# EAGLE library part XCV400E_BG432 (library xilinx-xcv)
xcv400e_bg432 edit this description Auto generated by make-symbol-device-package-bsdl.ulp Rev. 26 Source: xcv400e_bg432.bsd
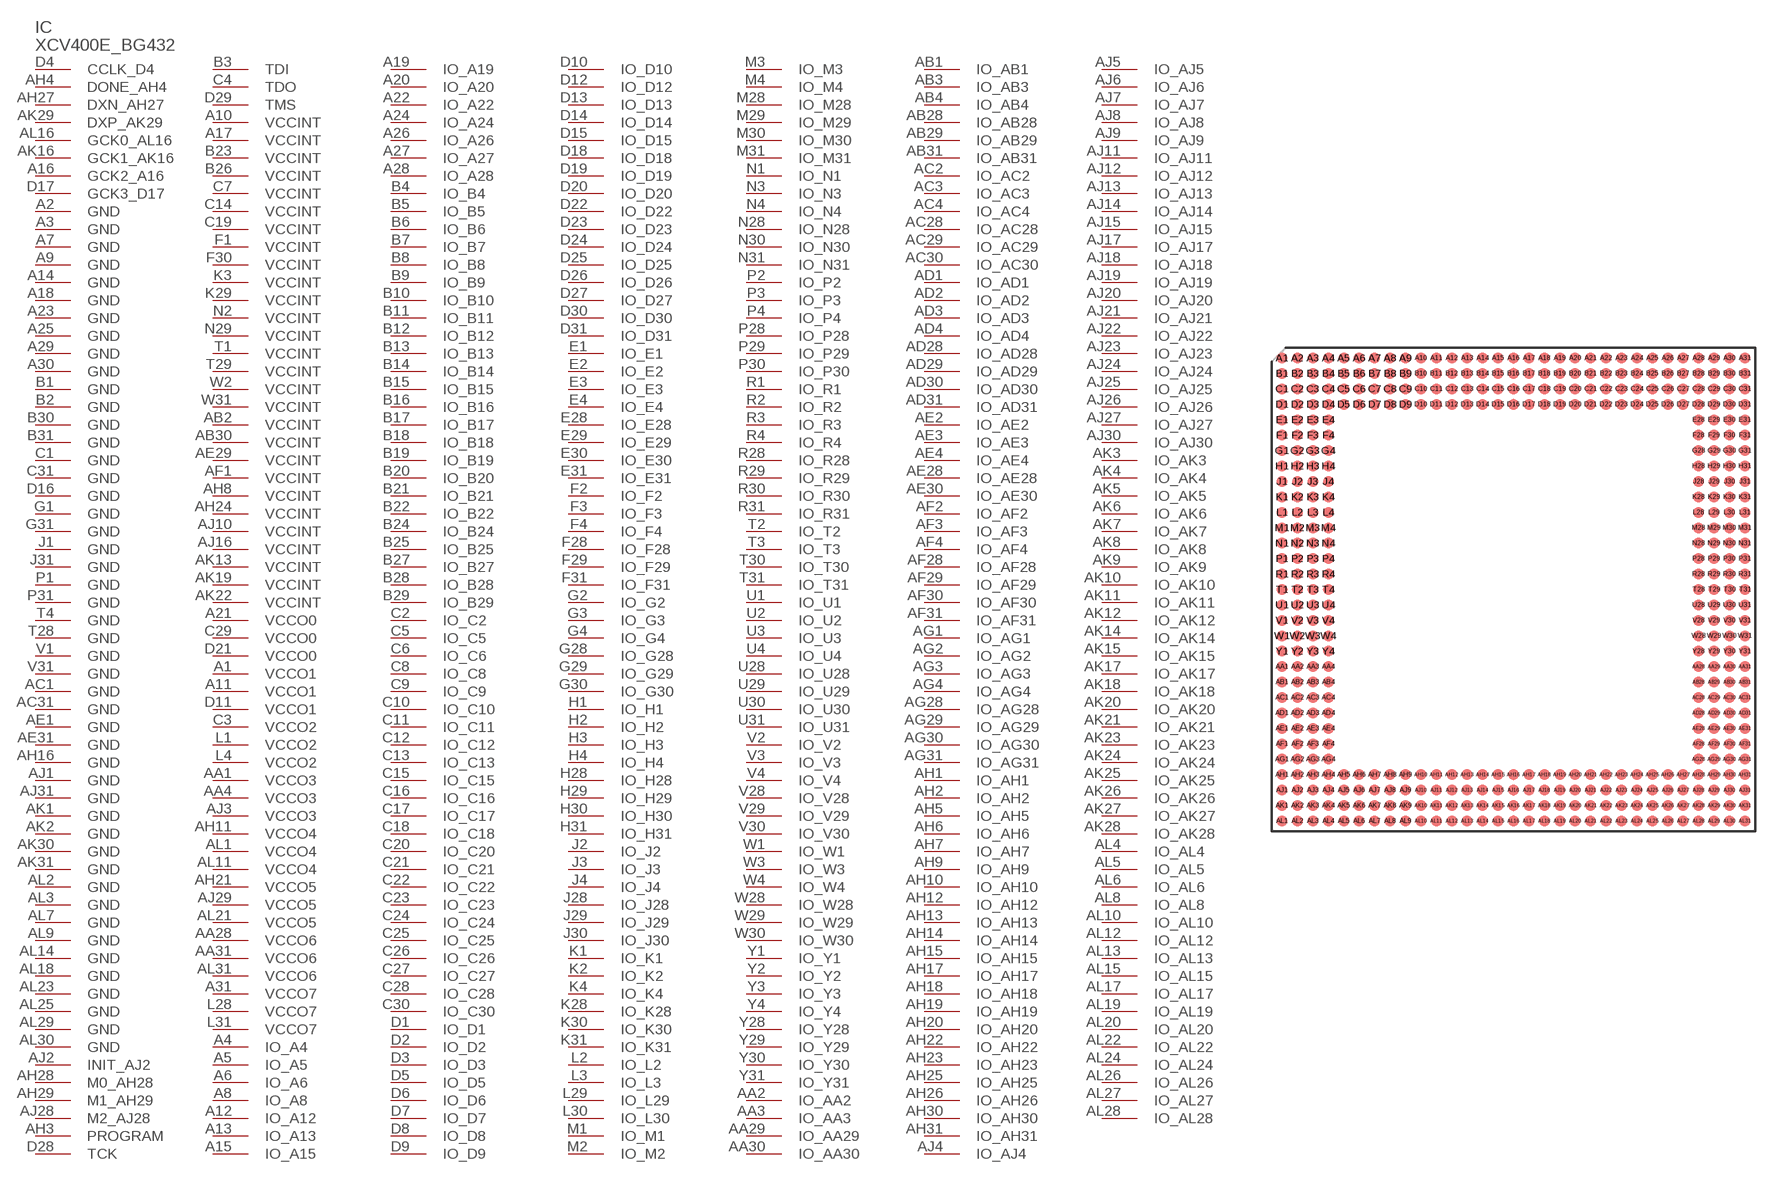
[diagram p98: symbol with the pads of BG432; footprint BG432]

Designator prefix IC

## XCV400E_BG432 (OC_FARNELL: unknown; OC_NEWARK: unknown)  [BG432]
A1  VCCO1  pwr
A2  GND  pwr
A3  GND  pwr
A4  IO_A4
A5  IO_A5
A6  IO_A6
A7  GND  pwr
A8  IO_A8
A9  GND  pwr
A10  VCCINT  pwr
A11  VCCO1  pwr
A12  IO_A12
A13  IO_A13
A14  GND  pwr
A15  IO_A15
A16  GCK2_A16  in
A17  VCCINT  pwr
A18  GND  pwr
A19  IO_A19
A20  IO_A20
A21  VCCO0  pwr
A22  IO_A22
A23  GND  pwr
A24  IO_A24
A25  GND  pwr
A26  IO_A26
A27  IO_A27
A28  IO_A28
A29  GND  pwr
A30  GND  pwr
A31  VCCO7  pwr
AA1  VCCO3  pwr
AA2  IO_AA2
AA3  IO_AA3
AA4  VCCO3  pwr
AA28  VCCO6  pwr
AA29  IO_AA29
AA30  IO_AA30
AA31  VCCO6  pwr
AB1  IO_AB1
AB2  VCCINT  pwr
AB3  IO_AB3
AB4  IO_AB4
AB28  IO_AB28
AB29  IO_AB29
AB30  VCCINT  pwr
AB31  IO_AB31
AC1  GND  pwr
AC2  IO_AC2
AC3  IO_AC3
AC4  IO_AC4
AC28  IO_AC28
AC29  IO_AC29
AC30  IO_AC30
AC31  GND  pwr
AD1  IO_AD1
AD2  IO_AD2
AD3  IO_AD3
AD4  IO_AD4
AD28  IO_AD28
AD29  IO_AD29
AD30  IO_AD30
AD31  IO_AD31
AE1  GND  pwr
AE2  IO_AE2
AE3  IO_AE3
AE4  IO_AE4
AE28  IO_AE28
AE29  VCCINT  pwr
AE30  IO_AE30
AE31  GND  pwr
AF1  VCCINT  pwr
AF2  IO_AF2
AF3  IO_AF3
AF4  IO_AF4
AF28  IO_AF28
AF29  IO_AF29
AF30  IO_AF30
AF31  IO_AF31
AG1  IO_AG1
AG2  IO_AG2
AG3  IO_AG3
AG4  IO_AG4
AG28  IO_AG28
AG29  IO_AG29
AG30  IO_AG30
AG31  IO_AG31
AH1  IO_AH1
AH2  IO_AH2
AH3  PROGRAM  in
AH4  DONE_AH4
AH5  IO_AH5
AH6  IO_AH6
AH7  IO_AH7
AH8  VCCINT  pwr
AH9  IO_AH9
AH10  IO_AH10
AH11  VCCO4  pwr
AH12  IO_AH12
AH13  IO_AH13
AH14  IO_AH14
AH15  IO_AH15
AH16  GND  pwr
AH17  IO_AH17
AH18  IO_AH18
AH19  IO_AH19
AH20  IO_AH20
AH21  VCCO5  pwr
AH22  IO_AH22
AH23  IO_AH23
AH24  VCCINT  pwr
AH25  IO_AH25
AH26  IO_AH26
AH27  DXN_AH27  pas
AH28  M0_AH28  in
AH29  M1_AH29  in
AH30  IO_AH30
AH31  IO_AH31
AJ1  GND  pwr
AJ2  INIT_AJ2
AJ3  VCCO3  pwr
AJ4  IO_AJ4
AJ5  IO_AJ5
AJ6  IO_AJ6
AJ7  IO_AJ7
AJ8  IO_AJ8
AJ9  IO_AJ9
AJ10  VCCINT  pwr
AJ11  IO_AJ11
AJ12  IO_AJ12
AJ13  IO_AJ13
AJ14  IO_AJ14
AJ15  IO_AJ15
AJ16  VCCINT  pwr
AJ17  IO_AJ17
AJ18  IO_AJ18
AJ19  IO_AJ19
AJ20  IO_AJ20
AJ21  IO_AJ21
AJ22  IO_AJ22
AJ23  IO_AJ23
AJ24  IO_AJ24
AJ25  IO_AJ25
AJ26  IO_AJ26
AJ27  IO_AJ27
AJ28  M2_AJ28  in
AJ29  VCCO5  pwr
AJ30  IO_AJ30
AJ31  GND  pwr
AK1  GND  pwr
AK2  GND  pwr
AK3  IO_AK3
AK4  IO_AK4
AK5  IO_AK5
AK6  IO_AK6
AK7  IO_AK7
AK8  IO_AK8
AK9  IO_AK9
AK10  IO_AK10
AK11  IO_AK11
AK12  IO_AK12
AK13  VCCINT  pwr
AK14  IO_AK14
AK15  IO_AK15
AK16  GCK1_AK16  in
AK17  IO_AK17
AK18  IO_AK18
AK19  VCCINT  pwr
AK20  IO_AK20
AK21  IO_AK21
AK22  VCCINT  pwr
AK23  IO_AK23
AK24  IO_AK24
AK25  IO_AK25
AK26  IO_AK26
AK27  IO_AK27
AK28  IO_AK28
AK29  DXP_AK29  pas
AK30  GND  pwr
AK31  GND  pwr
AL1  VCCO4  pwr
AL2  GND  pwr
AL3  GND  pwr
AL4  IO_AL4
AL5  IO_AL5
AL6  IO_AL6
AL7  GND  pwr
AL8  IO_AL8
AL9  GND  pwr
AL10  IO_AL10
AL11  VCCO4  pwr
AL12  IO_AL12
AL13  IO_AL13
AL14  GND  pwr
AL15  IO_AL15
AL16  GCK0_AL16  in
AL17  IO_AL17
AL18  GND  pwr
AL19  IO_AL19
AL20  IO_AL20
AL21  VCCO5  pwr
AL22  IO_AL22
AL23  GND  pwr
AL24  IO_AL24
AL25  GND  pwr
AL26  IO_AL26
AL27  IO_AL27
AL28  IO_AL28
AL29  GND  pwr
AL30  GND  pwr
AL31  VCCO6  pwr
B1  GND  pwr
B2  GND  pwr
B3  TDI  in
B4  IO_B4
B5  IO_B5
B6  IO_B6
B7  IO_B7
B8  IO_B8
B9  IO_B9
B10  IO_B10
B11  IO_B11
B12  IO_B12
B13  IO_B13
B14  IO_B14
B15  IO_B15
B16  IO_B16
B17  IO_B17
B18  IO_B18
B19  IO_B19
B20  IO_B20
B21  IO_B21
B22  IO_B22
B23  VCCINT  pwr
B24  IO_B24
B25  IO_B25
B26  VCCINT  pwr
B27  IO_B27
B28  IO_B28
B29  IO_B29
B30  GND  pwr
B31  GND  pwr
C1  GND  pwr
C2  IO_C2
C3  VCCO2  pwr
C4  TDO  out
C5  IO_C5
C6  IO_C6
C7  VCCINT  pwr
C8  IO_C8
C9  IO_C9
C10  IO_C10
C11  IO_C11
C12  IO_C12
C13  IO_C13
C14  VCCINT  pwr
C15  IO_C15
C16  IO_C16
C17  IO_C17
C18  IO_C18
C19  VCCINT  pwr
C20  IO_C20
C21  IO_C21
C22  IO_C22
C23  IO_C23
C24  IO_C24
C25  IO_C25
C26  IO_C26
C27  IO_C27
C28  IO_C28
C29  VCCO0  pwr
C30  IO_C30
C31  GND  pwr
D1  IO_D1
D2  IO_D2
D3  IO_D3
D4  CCLK_D4
D5  IO_D5
D6  IO_D6
D7  IO_D7
D8  IO_D8
D9  IO_D9
D10  IO_D10
D11  VCCO1  pwr
D12  IO_D12
D13  IO_D13
D14  IO_D14
D15  IO_D15
D16  GND  pwr
D17  GCK3_D17  in
D18  IO_D18
D19  IO_D19
D20  IO_D20
D21  VCCO0  pwr
D22  IO_D22
D23  IO_D23
D24  IO_D24
D25  IO_D25
D26  IO_D26
D27  IO_D27
D28  TCK  in
D29  TMS  in
D30  IO_D30
D31  IO_D31
E1  IO_E1
E2  IO_E2
E3  IO_E3
E4  IO_E4
E28  IO_E28
E29  IO_E29
E30  IO_E30
E31  IO_E31
F1  VCCINT  pwr
F2  IO_F2
F3  IO_F3
F4  IO_F4
F28  IO_F28
F29  IO_F29
F30  VCCINT  pwr
F31  IO_F31
G1  GND  pwr
G2  IO_G2
G3  IO_G3
G4  IO_G4
G28  IO_G28
G29  IO_G29
G30  IO_G30
G31  GND  pwr
H1  IO_H1
H2  IO_H2
H3  IO_H3
H4  IO_H4
H28  IO_H28
H29  IO_H29
H30  IO_H30
H31  IO_H31
J1  GND  pwr
J2  IO_J2
J3  IO_J3
J4  IO_J4
J28  IO_J28
J29  IO_J29
J30  IO_J30
J31  GND  pwr
K1  IO_K1
K2  IO_K2
K3  VCCINT  pwr
K4  IO_K4
K28  IO_K28
K29  VCCINT  pwr
K30  IO_K30
K31  IO_K31
L1  VCCO2  pwr
L2  IO_L2
L3  IO_L3
L4  VCCO2  pwr
L28  VCCO7  pwr
L29  IO_L29
L30  IO_L30
L31  VCCO7  pwr
M1  IO_M1
M2  IO_M2
M3  IO_M3
M4  IO_M4
M28  IO_M28
M29  IO_M29
M30  IO_M30
M31  IO_M31
N1  IO_N1
N2  VCCINT  pwr
N3  IO_N3
N4  IO_N4
N28  IO_N28
N29  VCCINT  pwr
N30  IO_N30
N31  IO_N31
P1  GND  pwr
P2  IO_P2
P3  IO_P3
P4  IO_P4
P28  IO_P28
P29  IO_P29
P30  IO_P30
P31  GND  pwr
R1  IO_R1
R2  IO_R2
R3  IO_R3
R4  IO_R4
R28  IO_R28
R29  IO_R29
R30  IO_R30
R31  IO_R31
T1  VCCINT  pwr
T2  IO_T2
T3  IO_T3
T4  GND  pwr
T28  GND  pwr
T29  VCCINT  pwr
T30  IO_T30
T31  IO_T31
U1  IO_U1
U2  IO_U2
U3  IO_U3
U4  IO_U4
U28  IO_U28
U29  IO_U29
U30  IO_U30
U31  IO_U31
V1  GND  pwr
V2  IO_V2
V3  IO_V3
V4  IO_V4
V28  IO_V28
V29  IO_V29
V30  IO_V30
V31  GND  pwr
W1  IO_W1
W2  VCCINT  pwr
W3  IO_W3
W4  IO_W4
W28  IO_W28
W29  IO_W29
W30  IO_W30
W31  VCCINT  pwr
Y1  IO_Y1
Y2  IO_Y2
Y3  IO_Y3
Y4  IO_Y4
Y28  IO_Y28
Y29  IO_Y29
Y30  IO_Y30
Y31  IO_Y31

## Footprint BG432 (pad centres in mm)
xcv300_bg432 edit this description Auto generated by make-symbol-device-package-bsdl.ulp Rev. 26 Source: xcv300_bg432.bsd
smd 0.9 x 0.9: A1 -19.05,19.05; A2 -17.78,19.05; A3 -16.51,19.05; A4 -15.24,19.05; A5 -13.97,19.05; A6 -12.7,19.05; A7 -11.43,19.05; A8 -10.16,19.05; A9 -8.89,19.05; A10 -7.62,19.05; A11 -6.35,19.05; A12 -5.08,19.05; A13 -3.81,19.05; A14 -2.54,19.05; A15 -1.27,19.05; A16 0,19.05; A17 1.27,19.05; A18 2.54,19.05; A19 3.81,19.05; A20 5.08,19.05; A21 6.35,19.05; A22 7.62,19.05; A23 8.89,19.05; A24 10.16,19.05; A25 11.43,19.05; A26 12.7,19.05; A27 13.97,19.05; A28 15.24,19.05; A29 16.51,19.05; A30 17.78,19.05; A31 19.05,19.05; AA1 -19.05,-6.35; AA2 -17.78,-6.35; AA3 -16.51,-6.35; AA4 -15.24,-6.35; AA28 15.24,-6.35; AA29 16.51,-6.35; AA30 17.78,-6.35; AA31 19.05,-6.35; AB1 -19.05,-7.62; AB2 -17.78,-7.62; AB3 -16.51,-7.62; AB4 -15.24,-7.62; AB28 15.24,-7.62; AB29 16.51,-7.62; AB30 17.78,-7.62; AB31 19.05,-7.62; AC1 -19.05,-8.89; AC2 -17.78,-8.89; AC3 -16.51,-8.89; AC4 -15.24,-8.89; AC28 15.24,-8.89; AC29 16.51,-8.89; AC30 17.78,-8.89; AC31 19.05,-8.89; AD1 -19.05,-10.16; AD2 -17.78,-10.16; AD3 -16.51,-10.16; AD4 -15.24,-10.16; AD28 15.24,-10.16; AD29 16.51,-10.16; AD30 17.78,-10.16; AD31 19.05,-10.16; AE1 -19.05,-11.43; AE2 -17.78,-11.43; AE3 -16.51,-11.43; AE4 -15.24,-11.43; AE28 15.24,-11.43; AE29 16.51,-11.43; AE30 17.78,-11.43; AE31 19.05,-11.43; AF1 -19.05,-12.7; AF2 -17.78,-12.7; AF3 -16.51,-12.7; AF4 -15.24,-12.7; AF28 15.24,-12.7; AF29 16.51,-12.7; AF30 17.78,-12.7; AF31 19.05,-12.7; AG1 -19.05,-13.97; AG2 -17.78,-13.97; AG3 -16.51,-13.97; AG4 -15.24,-13.97; AG28 15.24,-13.97; AG29 16.51,-13.97; AG30 17.78,-13.97; AG31 19.05,-13.97; AH1 -19.05,-15.24; AH2 -17.78,-15.24; AH3 -16.51,-15.24; AH4 -15.24,-15.24; AH5 -13.97,-15.24; AH6 -12.7,-15.24; AH7 -11.43,-15.24; AH8 -10.16,-15.24; AH9 -8.89,-15.24; AH10 -7.62,-15.24; AH11 -6.35,-15.24; AH12 -5.08,-15.24; AH13 -3.81,-15.24; AH14 -2.54,-15.24; AH15 -1.27,-15.24; AH16 0,-15.24; AH17 1.27,-15.24; AH18 2.54,-15.24; AH19 3.81,-15.24; AH20 5.08,-15.24; AH21 6.35,-15.24; AH22 7.62,-15.24; AH23 8.89,-15.24; AH24 10.16,-15.24; AH25 11.43,-15.24; AH26 12.7,-15.24; AH27 13.97,-15.24; AH28 15.24,-15.24; AH29 16.51,-15.24; AH30 17.78,-15.24; AH31 19.05,-15.24; AJ1 -19.05,-16.51; AJ2 -17.78,-16.51; AJ3 -16.51,-16.51; AJ4 -15.24,-16.51; AJ5 -13.97,-16.51; AJ6 -12.7,-16.51; AJ7 -11.43,-16.51; AJ8 -10.16,-16.51; AJ9 -8.89,-16.51; AJ10 -7.62,-16.51; AJ11 -6.35,-16.51; AJ12 -5.08,-16.51; AJ13 -3.81,-16.51; AJ14 -2.54,-16.51; AJ15 -1.27,-16.51; AJ16 0,-16.51; AJ17 1.27,-16.51; AJ18 2.54,-16.51; AJ19 3.81,-16.51; AJ20 5.08,-16.51; AJ21 6.35,-16.51; AJ22 7.62,-16.51; AJ23 8.89,-16.51; AJ24 10.16,-16.51; AJ25 11.43,-16.51; AJ26 12.7,-16.51; AJ27 13.97,-16.51; AJ28 15.24,-16.51; AJ29 16.51,-16.51; AJ30 17.78,-16.51; AJ31 19.05,-16.51; AK1 -19.05,-17.78; AK2 -17.78,-17.78; AK3 -16.51,-17.78; AK4 -15.24,-17.78; AK5 -13.97,-17.78; AK6 -12.7,-17.78; AK7 -11.43,-17.78; AK8 -10.16,-17.78; AK9 -8.89,-17.78; AK10 -7.62,-17.78; AK11 -6.35,-17.78; AK12 -5.08,-17.78; AK13 -3.81,-17.78; AK14 -2.54,-17.78; AK15 -1.27,-17.78; AK16 0,-17.78; AK17 1.27,-17.78; AK18 2.54,-17.78; AK19 3.81,-17.78; AK20 5.08,-17.78; AK21 6.35,-17.78; AK22 7.62,-17.78; AK23 8.89,-17.78; AK24 10.16,-17.78; AK25 11.43,-17.78; AK26 12.7,-17.78; AK27 13.97,-17.78; AK28 15.24,-17.78; AK29 16.51,-17.78; AK30 17.78,-17.78; AK31 19.05,-17.78; AL1 -19.05,-19.05; AL2 -17.78,-19.05; AL3 -16.51,-19.05; AL4 -15.24,-19.05; AL5 -13.97,-19.05; AL6 -12.7,-19.05; AL7 -11.43,-19.05; AL8 -10.16,-19.05; AL9 -8.89,-19.05; AL10 -7.62,-19.05; AL11 -6.35,-19.05; AL12 -5.08,-19.05; AL13 -3.81,-19.05; AL14 -2.54,-19.05; AL15 -1.27,-19.05; AL16 0,-19.05; AL17 1.27,-19.05; AL18 2.54,-19.05; AL19 3.81,-19.05; AL20 5.08,-19.05; AL21 6.35,-19.05; AL22 7.62,-19.05; AL23 8.89,-19.05; AL24 10.16,-19.05; AL25 11.43,-19.05; AL26 12.7,-19.05; AL27 13.97,-19.05; AL28 15.24,-19.05; AL29 16.51,-19.05; AL30 17.78,-19.05; AL31 19.05,-19.05; B1 -19.05,17.78; B2 -17.78,17.78; B3 -16.51,17.78; B4 -15.24,17.78; B5 -13.97,17.78; B6 -12.7,17.78; B7 -11.43,17.78; B8 -10.16,17.78; B9 -8.89,17.78; B10 -7.62,17.78; B11 -6.35,17.78; B12 -5.08,17.78; B13 -3.81,17.78; B14 -2.54,17.78; B15 -1.27,17.78; B16 0,17.78; B17 1.27,17.78; B18 2.54,17.78; B19 3.81,17.78; B20 5.08,17.78; B21 6.35,17.78; B22 7.62,17.78; B23 8.89,17.78; B24 10.16,17.78; B25 11.43,17.78; B26 12.7,17.78; B27 13.97,17.78; B28 15.24,17.78; B29 16.51,17.78; B30 17.78,17.78; B31 19.05,17.78; C1 -19.05,16.51; C2 -17.78,16.51; C3 -16.51,16.51; C4 -15.24,16.51; C5 -13.97,16.51; C6 -12.7,16.51; C7 -11.43,16.51; C8 -10.16,16.51; C9 -8.89,16.51; C10 -7.62,16.51; C11 -6.35,16.51; C12 -5.08,16.51; C13 -3.81,16.51; C14 -2.54,16.51; C15 -1.27,16.51; C16 0,16.51; C17 1.27,16.51; C18 2.54,16.51; C19 3.81,16.51; C20 5.08,16.51; C21 6.35,16.51; C22 7.62,16.51; C23 8.89,16.51; C24 10.16,16.51; C25 11.43,16.51; C26 12.7,16.51; C27 13.97,16.51; C28 15.24,16.51; C29 16.51,16.51; C30 17.78,16.51; C31 19.05,16.51; D1 -19.05,15.24; D2 -17.78,15.24; D3 -16.51,15.24; D4 -15.24,15.24; D5 -13.97,15.24; D6 -12.7,15.24; D7 -11.43,15.24; D8 -10.16,15.24; D9 -8.89,15.24; D10 -7.62,15.24; D11 -6.35,15.24; D12 -5.08,15.24; D13 -3.81,15.24; D14 -2.54,15.24; D15 -1.27,15.24; D16 0,15.24; D17 1.27,15.24; D18 2.54,15.24; D19 3.81,15.24; D20 5.08,15.24; D21 6.35,15.24; D22 7.62,15.24; D23 8.89,15.24; D24 10.16,15.24; D25 11.43,15.24; D26 12.7,15.24; D27 13.97,15.24; D28 15.24,15.24; D29 16.51,15.24; D30 17.78,15.24; D31 19.05,15.24; E1 -19.05,13.97; E2 -17.78,13.97; E3 -16.51,13.97; E4 -15.24,13.97; E28 15.24,13.97; E29 16.51,13.97; E30 17.78,13.97; E31 19.05,13.97; F1 -19.05,12.7; F2 -17.78,12.7; F3 -16.51,12.7; F4 -15.24,12.7; F28 15.24,12.7; F29 16.51,12.7; F30 17.78,12.7; F31 19.05,12.7; G1 -19.05,11.43; G2 -17.78,11.43; G3 -16.51,11.43; G4 -15.24,11.43; G28 15.24,11.43; G29 16.51,11.43; G30 17.78,11.43; G31 19.05,11.43; H1 -19.05,10.16; H2 -17.78,10.16; H3 -16.51,10.16; H4 -15.24,10.16; H28 15.24,10.16; H29 16.51,10.16; H30 17.78,10.16; H31 19.05,10.16; J1 -19.05,8.89; J2 -17.78,8.89; J3 -16.51,8.89; J4 -15.24,8.89; J28 15.24,8.89; J29 16.51,8.89; J30 17.78,8.89; J31 19.05,8.89; K1 -19.05,7.62; K2 -17.78,7.62; K3 -16.51,7.62; K4 -15.24,7.62; K28 15.24,7.62; K29 16.51,7.62; K30 17.78,7.62; K31 19.05,7.62; L1 -19.05,6.35; L2 -17.78,6.35; L3 -16.51,6.35; L4 -15.24,6.35; L28 15.24,6.35; L29 16.51,6.35; L30 17.78,6.35; L31 19.05,6.35; M1 -19.05,5.08; M2 -17.78,5.08; M3 -16.51,5.08; M4 -15.24,5.08; M28 15.24,5.08; M29 16.51,5.08; M30 17.78,5.08; M31 19.05,5.08; N1 -19.05,3.81; N2 -17.78,3.81; N3 -16.51,3.81; N4 -15.24,3.81; N28 15.24,3.81; N29 16.51,3.81; N30 17.78,3.81; N31 19.05,3.81; P1 -19.05,2.54; P2 -17.78,2.54; P3 -16.51,2.54; P4 -15.24,2.54; P28 15.24,2.54; P29 16.51,2.54; P30 17.78,2.54; P31 19.05,2.54; R1 -19.05,1.27; R2 -17.78,1.27; R3 -16.51,1.27; R4 -15.24,1.27; R28 15.24,1.27; R29 16.51,1.27; R30 17.78,1.27; R31 19.05,1.27; T1 -19.05,0; T2 -17.78,0; T3 -16.51,0; T4 -15.24,0; T28 15.24,0; T29 16.51,0; T30 17.78,0; T31 19.05,0; U1 -19.05,-1.27; U2 -17.78,-1.27; U3 -16.51,-1.27; U4 -15.24,-1.27; U28 15.24,-1.27; U29 16.51,-1.27; U30 17.78,-1.27; U31 19.05,-1.27; V1 -19.05,-2.54; V2 -17.78,-2.54; V3 -16.51,-2.54; V4 -15.24,-2.54; V28 15.24,-2.54; V29 16.51,-2.54; V30 17.78,-2.54; V31 19.05,-2.54; W1 -19.05,-3.81; W2 -17.78,-3.81; W3 -16.51,-3.81; W4 -15.24,-3.81; W28 15.24,-3.81; W29 16.51,-3.81; W30 17.78,-3.81; W31 19.05,-3.81; Y1 -19.05,-5.08; Y2 -17.78,-5.08; Y3 -16.51,-5.08; Y4 -15.24,-5.08; Y28 15.24,-5.08; Y29 16.51,-5.08; Y30 17.78,-5.08; Y31 19.05,-5.08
